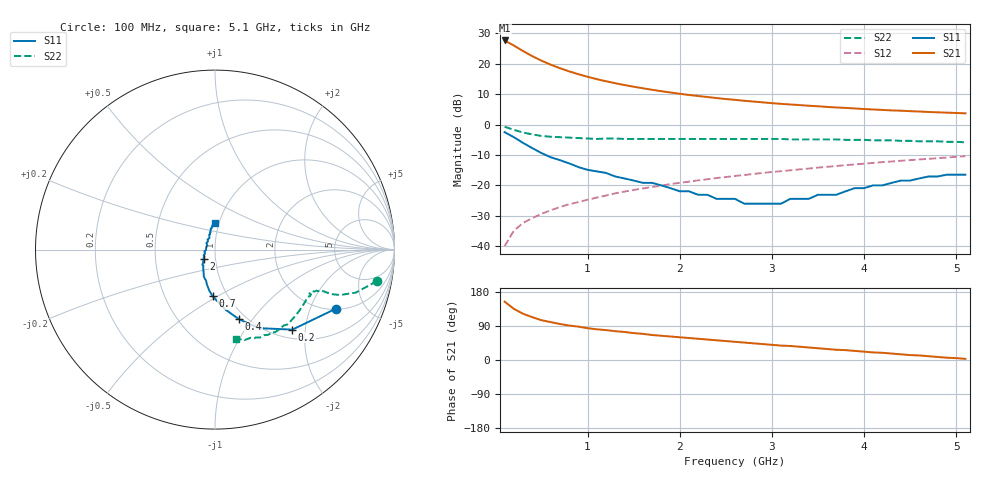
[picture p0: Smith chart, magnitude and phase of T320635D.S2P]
!AT-32063
!S PARAMETERS per side at Vce=5 V  Ic=10mA.  LAST UPDATED 08-19-96
# ghz s ma r 50
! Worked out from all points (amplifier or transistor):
!   51 points, 100 MHz to 5.1 GHz, reference 50 ohm
!   highest |S21| = 27.7 dB at 100 MHz (marker M1)
!   |S21| within 3 dB of that: start of sweep to 273.4 MHz
!   unconditionally stable (mu >= 1): 863.5 MHz to 3.826 GHz
!   at 900 MHz: K = 1.02, MAG = 20.3 dB, |S12| = -25.5 dB
!   at 2.6 GHz: K = 1.06, MAG = 11.0 dB, |S12| = -16.9 dB
!   at 5.1 GHz: K = 0.94, MSG = 7.0 dB, |S12| = -10.4 dB
!   S11 on the Smith chart (normalised r, x): 100 MHz: 2.04, -3.07; 200 MHz: 1.18, -1.71; 400 MHz: 0.92, -0.86; 700 MHz: 0.85, -0.47; 2 GHz: 0.88, -0.09; 5.1 GHz: 0.96, +0.29
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0.1  0.75 -26.0  24.17 154.0  0.01 77.0  0.92 -11.0
0.2  0.62 -46.0  19.94 135.0  0.018 70.0  0.82 -17.0
0.3  0.5 -61.0  16.19 122.0  0.024 67.0  0.74 -20.0
0.4  0.41 -71.0  13.35 113.0  0.029 66.0  0.69 -21.0
0.5  0.34 -80.0  11.25 105.0  0.034 66.0  0.65 -21.0
0.6  0.29 -87.0  9.66 100.0  0.039 66.0  0.63 -21.0
0.7  0.26 -93.0  8.46 95.0  0.044 66.0  0.62 -22.0
0.8  0.23 -98.0  7.5 91.0  0.049 67.0  0.61 -22.0
0.9  0.2 -103.0  6.74 88.0  0.053 67.0  0.6 -23.0
1  0.18 -106.0  6.11 84.0  0.058 67.0  0.59 -23.0
1.1  0.17 -110.0  5.58 81.0  0.063 67.0  0.58 -25.0
1.3  0.14 -117.0  4.79 76.0  0.074 66.0  0.59 -26.0
1.5  0.12 -123.0  4.19 71.0  0.084 66.0  0.58 -28.0
1.8  0.1 -132.0  3.54 64.0  0.099 64.0  0.58 -31.0
2  0.08 -140.0  3.21 60.0  0.11 63.0  0.58 -33.0
2.6  0.06 -170.0  2.55 48.0  0.143 59.0  0.58 -40.0
2.7  0.05 -177.0  2.46 46.0  0.148 58.0  0.58 -42.0
3.1  0.05 149.0  2.19 38.0  0.171 55.0  0.58 -46.0
3.5  0.07 126.0  2 31.0  0.196 51.0  0.57 -51.0
3.7  0.07 117.0  1.91 27.0  0.208 49.0  0.57 -54.0
4.3  0.11 103.0  1.71 17.0  0.247 43.0  0.55 -63.0
5.1  0.15 89.0  1.53 3.0  0.302 34.0  0.51 -77.0
